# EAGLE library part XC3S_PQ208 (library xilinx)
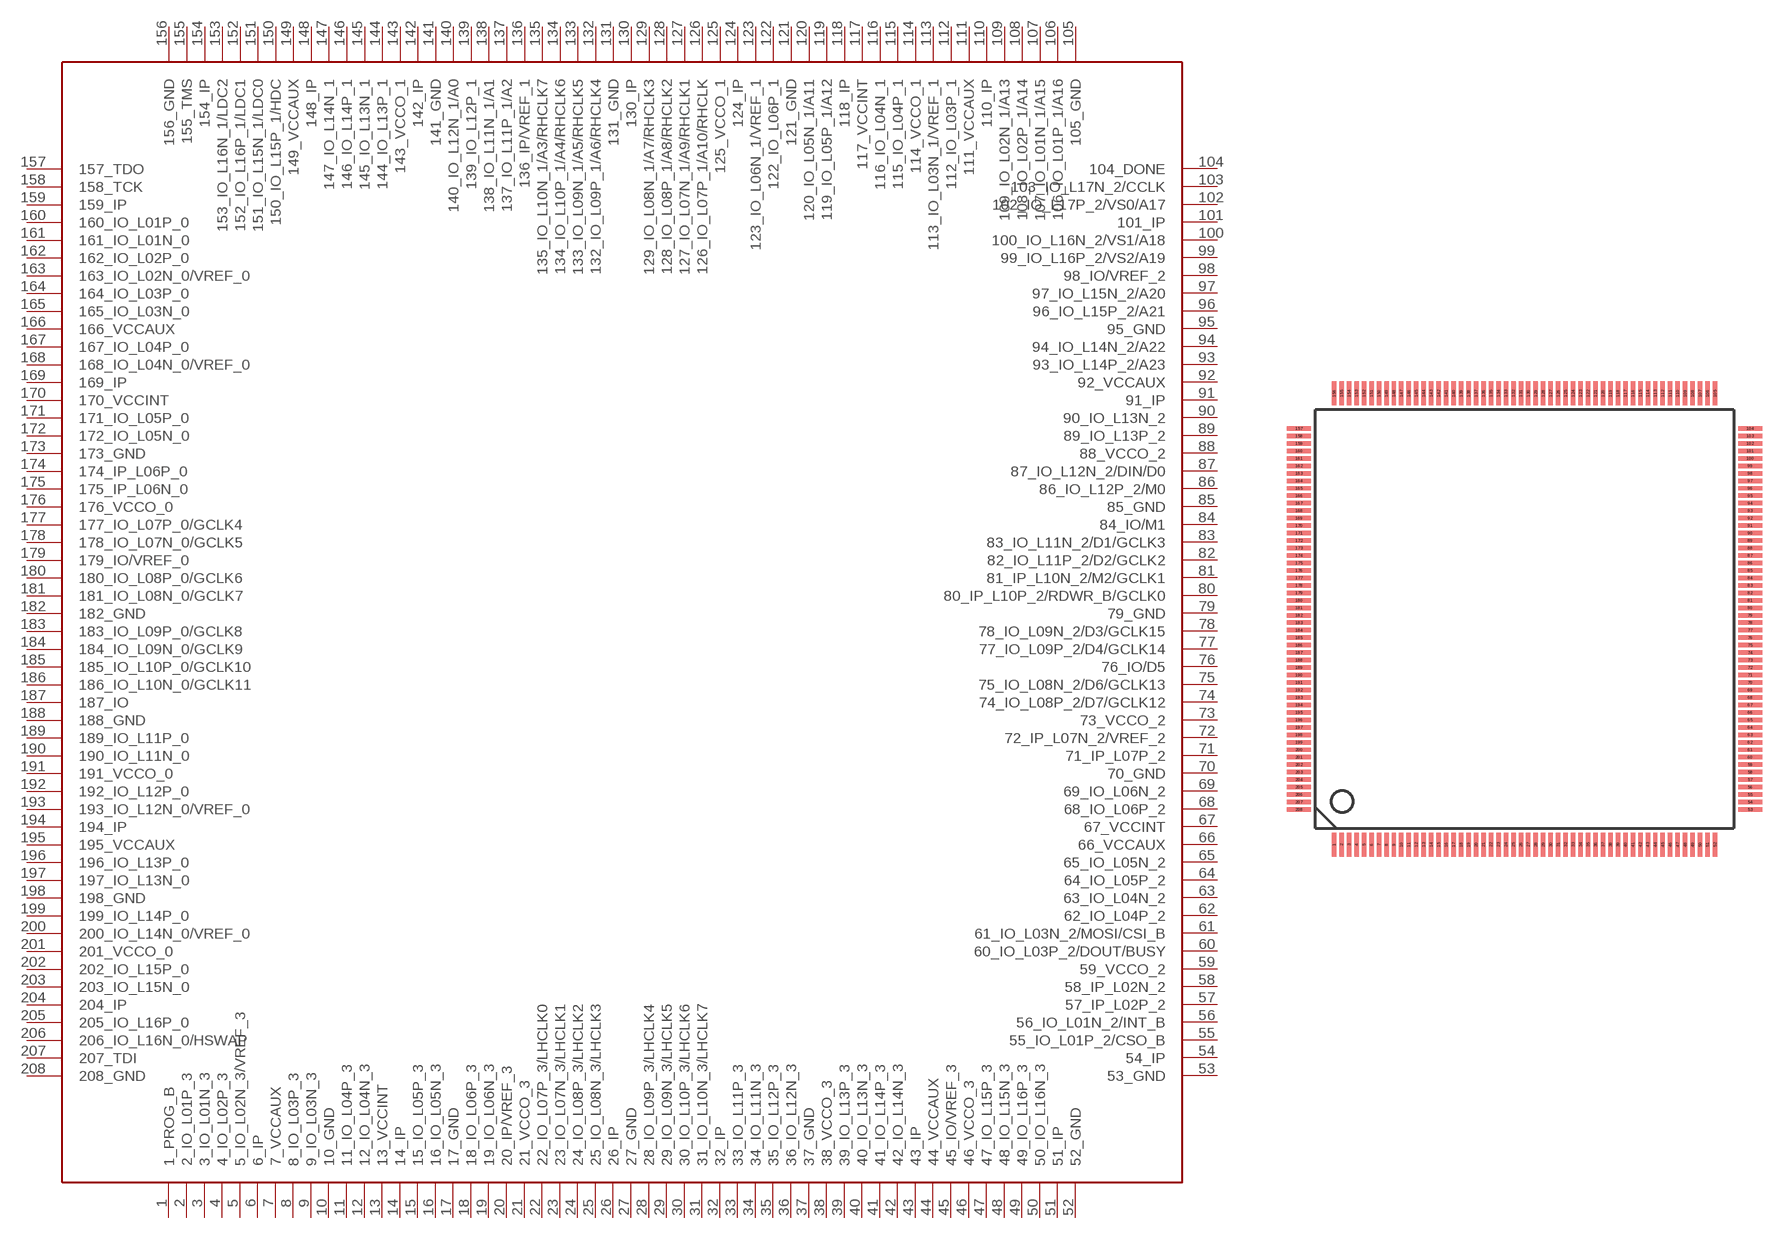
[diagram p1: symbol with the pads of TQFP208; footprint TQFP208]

Designator prefix U

## XC3S_PQ208  [TQFP208]
1  1_PROG_B
2  2_IO_L01P_3
3  3_IO_L01N_3
4  4_IO_L02P_3
5  5_IO_L02N_3/VREF_3
6  6_IP
7  7_VCCAUX
8  8_IO_L03P_3
9  9_IO_L03N_3
10  10_GND
11  11_IO_L04P_3
12  12_IO_L04N_3
13  13_VCCINT
14  14_IP
15  15_IO_L05P_3
16  16_IO_L05N_3
17  17_GND
18  18_IO_L06P_3
19  19_IO_L06N_3
20  20_IP/VREF_3
21  21_VCCO_3
22  22_IO_L07P_3/LHCLK0
23  23_IO_L07N_3/LHCLK1
24  24_IO_L08P_3/LHCLK2
25  25_IO_L08N_3/LHCLK3
26  26_IP
27  27_GND
28  28_IO_L09P_3/LHCLK4
29  29_IO_L09N_3/LHCLK5
30  30_IO_L10P_3/LHCLK6
31  31_IO_L10N_3/LHCLK7
32  32_IP
33  33_IO_L11P_3
34  34_IO_L11N_3
35  35_IO_L12P_3
36  36_IO_L12N_3
37  37_GND
38  38_VCCO_3
39  39_IO_L13P_3
40  40_IO_L13N_3
41  41_IO_L14P_3
42  42_IO_L14N_3
43  43_IP
44  44_VCCAUX
45  45_IO/VREF_3
46  46_VCCO_3
47  47_IO_L15P_3
48  48_IO_L15N_3
49  49_IO_L16P_3
50  50_IO_L16N_3
51  51_IP
52  52_GND
53  53_GND
54  54_IP
55  55_IO_L01P_2/CSO_B
56  56_IO_L01N_2/INT_B
57  57_IP_L02P_2
58  58_IP_L02N_2
59  59_VCCO_2
60  60_IO_L03P_2/DOUT/BUSY
61  61_IO_L03N_2/MOSI/CSI_B
62  62_IO_L04P_2
63  63_IO_L04N_2
64  64_IO_L05P_2
65  65_IO_L05N_2
66  66_VCCAUX
67  67_VCCINT
68  68_IO_L06P_2
69  69_IO_L06N_2
70  70_GND
71  71_IP_L07P_2
72  72_IP_L07N_2/VREF_2
73  73_VCCO_2
74  74_IO_L08P_2/D7/GCLK12
75  75_IO_L08N_2/D6/GCLK13
76  76_IO/D5
77  77_IO_L09P_2/D4/GCLK14
78  78_IO_L09N_2/D3/GCLK15
79  79_GND
80  80_IP_L10P_2/RDWR_B/GCLK0
81  81_IP_L10N_2/M2/GCLK1
82  82_IO_L11P_2/D2/GCLK2
83  83_IO_L11N_2/D1/GCLK3
84  84_IO/M1
85  85_GND
86  86_IO_L12P_2/M0
87  87_IO_L12N_2/DIN/D0
88  88_VCCO_2
89  89_IO_L13P_2
90  90_IO_L13N_2
91  91_IP
92  92_VCCAUX
93  93_IO_L14P_2/A23
94  94_IO_L14N_2/A22
95  95_GND
96  96_IO_L15P_2/A21
97  97_IO_L15N_2/A20
98  98_IO/VREF_2
99  99_IO_L16P_2/VS2/A19
100  100_IO_L16N_2/VS1/A18
101  101_IP
102  102_IO_L17P_2/VS0/A17
103  103_IO_L17N_2/CCLK
104  104_DONE
105  105_GND
106  106_IO_L01P_1/A16
107  107_IO_L01N_1/A15
108  108_IO_L02P_1/A14
109  109_IO_L02N_1/A13
110  110_IP
111  111_VCCAUX
112  112_IO_L03P_1
113  113_IO_L03N_1/VREF_1
114  114_VCCO_1
115  115_IO_L04P_1
116  116_IO_L04N_1
117  117_VCCINT
118  118_IP
119  119_IO_L05P_1/A12
120  120_IO_L05N_1/A11
121  121_GND
122  122_IO_L06P_1
123  123_IO_L06N_1/VREF_1
124  124_IP
125  125_VCCO_1
126  126_IO_L07P_1/A10/RHCLK
127  127_IO_L07N_1/A9/RHCLK1
128  128_IO_L08P_1/A8/RHCLK2
129  129_IO_L08N_1/A7/RHCLK3
130  130_IP
131  131_GND
132  132_IO_L09P_1/A6/RHCLK4
133  133_IO_L09N_1/A5/RHCLK5
134  134_IO_L10P_1/A4/RHCLK6
135  135_IO_L10N_1/A3/RHCLK7
136  136_IP/VREF_1
137  137_IO_L11P_1/A2
138  138_IO_L11N_1/A1
139  139_IO_L12P_1
140  140_IO_L12N_1/A0
141  141_GND
142  142_IP
143  143_VCCO_1
144  144_IO_L13P_1
145  145_IO_L13N_1
146  146_IO_L14P_1
147  147_IO_L14N_1
148  148_IP
149  149_VCCAUX
150  150_IO_L15P_1/HDC
151  151_IO_L15N_1/LDC0
152  152_IO_L16P_1/LDC1
153  153_IO_L16N_1/LDC2
154  154_IP
155  155_TMS
156  156_GND
157  157_TDO
158  158_TCK
159  159_IP
160  160_IO_L01P_0
161  161_IO_L01N_0
162  162_IO_L02P_0
163  163_IO_L02N_0/VREF_0
164  164_IO_L03P_0
165  165_IO_L03N_0
166  166_VCCAUX
167  167_IO_L04P_0
168  168_IO_L04N_0/VREF_0
169  169_IP
170  170_VCCINT
171  171_IO_L05P_0
172  172_IO_L05N_0
173  173_GND
174  174_IP_L06P_0
175  175_IP_L06N_0
176  176_VCCO_0
177  177_IO_L07P_0/GCLK4
178  178_IO_L07N_0/GCLK5
179  179_IO/VREF_0
180  180_IO_L08P_0/GCLK6
181  181_IO_L08N_0/GCLK7
182  182_GND
183  183_IO_L09P_0/GCLK8
184  184_IO_L09N_0/GCLK9
185  185_IO_L10P_0/GCLK10
186  186_IO_L10N_0/GCLK11
187  187_IO
188  188_GND
189  189_IO_L11P_0
190  190_IO_L11N_0
191  191_VCCO_0
192  192_IO_L12P_0
193  193_IO_L12N_0/VREF_0
194  194_IP
195  195_VCCAUX
196  196_IO_L13P_0
197  197_IO_L13N_0
198  198_GND
199  199_IO_L14P_0
200  200_IO_L14N_0/VREF_0
201  201_VCCO_0
202  202_IO_L15P_0
203  203_IO_L15N_0
204  204_IP
205  205_IO_L16P_0
206  206_IO_L16N_0/HSWAP
207  207_TDI
208  208_GND

## Footprint TQFP208 (pad centres in mm)
smd 0.3 x 1.6: 1 -12.75,-15.1; 2 -12.25,-15.1; 3 -11.75,-15.1; 4 -11.25,-15.1; 5 -10.75,-15.1; 6 -10.25,-15.1; 7 -9.75,-15.1; 8 -9.25,-15.1; 9 -8.75,-15.1; 10 -8.25,-15.1; 11 -7.75,-15.1; 12 -7.25,-15.1; 13 -6.75,-15.1; 14 -6.25,-15.1; 15 -5.75,-15.1; 16 -5.25,-15.1; 17 -4.75,-15.1; 18 -4.25,-15.1; 19 -3.75,-15.1; 20 -3.25,-15.1; 21 -2.75,-15.1; 22 -2.25,-15.1; 23 -1.75,-15.1; 24 -1.25,-15.1; 25 -0.75,-15.1; 26 -0.25,-15.1; 27 0.25,-15.1; 28 0.75,-15.1; 29 1.25,-15.1; 30 1.75,-15.1; 31 2.25,-15.1; 32 2.75,-15.1; 33 3.25,-15.1; 34 3.75,-15.1; 35 4.25,-15.1; 36 4.75,-15.1; 37 5.25,-15.1; 38 5.75,-15.1; 39 6.25,-15.1; 40 6.75,-15.1; 41 7.25,-15.1; 42 7.75,-15.1; 43 8.25,-15.1; 44 8.75,-15.1; 45 9.25,-15.1; 46 9.75,-15.1; 47 10.25,-15.1; 48 10.75,-15.1; 49 11.25,-15.1; 50 11.75,-15.1; 51 12.25,-15.1; 52 12.75,-15.1; 105 12.75,15.1; 106 12.25,15.1; 107 11.75,15.1; 108 11.25,15.1; 109 10.75,15.1; 110 10.25,15.1; 111 9.75,15.1; 112 9.25,15.1; 113 8.75,15.1; 114 8.25,15.1; 115 7.75,15.1; 116 7.25,15.1; 117 6.75,15.1; 118 6.25,15.1; 119 5.75,15.1; 120 5.25,15.1; 121 4.75,15.1; 122 4.25,15.1; 123 3.75,15.1; 124 3.25,15.1; 125 2.75,15.1; 126 2.25,15.1; 127 1.75,15.1; 128 1.25,15.1; 129 0.75,15.1; 130 0.25,15.1; 131 -0.25,15.1; 132 -0.75,15.1; 133 -1.25,15.1; 134 -1.75,15.1; 135 -2.25,15.1; 136 -2.75,15.1; 137 -3.25,15.1; 138 -3.75,15.1; 139 -4.25,15.1; 140 -4.75,15.1; 141 -5.25,15.1; 142 -5.75,15.1; 143 -6.25,15.1; 144 -6.75,15.1; 145 -7.25,15.1; 146 -7.75,15.1; 147 -8.25,15.1; 148 -8.75,15.1; 149 -9.25,15.1; 150 -9.75,15.1; 151 -10.25,15.1; 152 -10.75,15.1; 153 -11.25,15.1; 154 -11.75,15.1; 155 -12.25,15.1; 156 -12.75,15.1
smd 1.6 x 0.3: 53 15.1,-12.75; 54 15.1,-12.25; 55 15.1,-11.75; 56 15.1,-11.25; 57 15.1,-10.75; 58 15.1,-10.25; 59 15.1,-9.75; 60 15.1,-9.25; 61 15.1,-8.75; 62 15.1,-8.25; 63 15.1,-7.75; 64 15.1,-7.25; 65 15.1,-6.75; 66 15.1,-6.25; 67 15.1,-5.75; 68 15.1,-5.25; 69 15.1,-4.75; 70 15.1,-4.25; 71 15.1,-3.75; 72 15.1,-3.25; 73 15.1,-2.75; 74 15.1,-2.25; 75 15.1,-1.75; 76 15.1,-1.25; 77 15.1,-0.75; 78 15.1,-0.25; 79 15.1,0.25; 80 15.1,0.75; 81 15.1,1.25; 82 15.1,1.75; 83 15.1,2.25; 84 15.1,2.75; 85 15.1,3.25; 86 15.1,3.75; 87 15.1,4.25; 88 15.1,4.75; 89 15.1,5.25; 90 15.1,5.75; 91 15.1,6.25; 92 15.1,6.75; 93 15.1,7.25; 94 15.1,7.75; 95 15.1,8.25; 96 15.1,8.75; 97 15.1,9.25; 98 15.1,9.75; 99 15.1,10.25; 100 15.1,10.75; 101 15.1,11.25; 102 15.1,11.75; 103 15.1,12.25; 104 15.1,12.75; 157 -15.1,12.75; 158 -15.1,12.25; 159 -15.1,11.75; 160 -15.1,11.25; 161 -15.1,10.75; 162 -15.1,10.25; 163 -15.1,9.75; 164 -15.1,9.25; 165 -15.1,8.75; 166 -15.1,8.25; 167 -15.1,7.75; 168 -15.1,7.25; 169 -15.1,6.75; 170 -15.1,6.25; 171 -15.1,5.75; 172 -15.1,5.25; 173 -15.1,4.75; 174 -15.1,4.25; 175 -15.1,3.75; 176 -15.1,3.25; 177 -15.1,2.75; 178 -15.1,2.25; 179 -15.1,1.75; 180 -15.1,1.25; 181 -15.1,0.75; 182 -15.1,0.25; 183 -15.1,-0.25; 184 -15.1,-0.75; 185 -15.1,-1.25; 186 -15.1,-1.75; 187 -15.1,-2.25; 188 -15.1,-2.75; 189 -15.1,-3.25; 190 -15.1,-3.75; 191 -15.1,-4.25; 192 -15.1,-4.75; 193 -15.1,-5.25; 194 -15.1,-5.75; 195 -15.1,-6.25; 196 -15.1,-6.75; 197 -15.1,-7.25; 198 -15.1,-7.75; 199 -15.1,-8.25; 200 -15.1,-8.75; 201 -15.1,-9.25; 202 -15.1,-9.75; 203 -15.1,-10.25; 204 -15.1,-10.75; 205 -15.1,-11.25; 206 -15.1,-11.75; 207 -15.1,-12.25; 208 -15.1,-12.75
